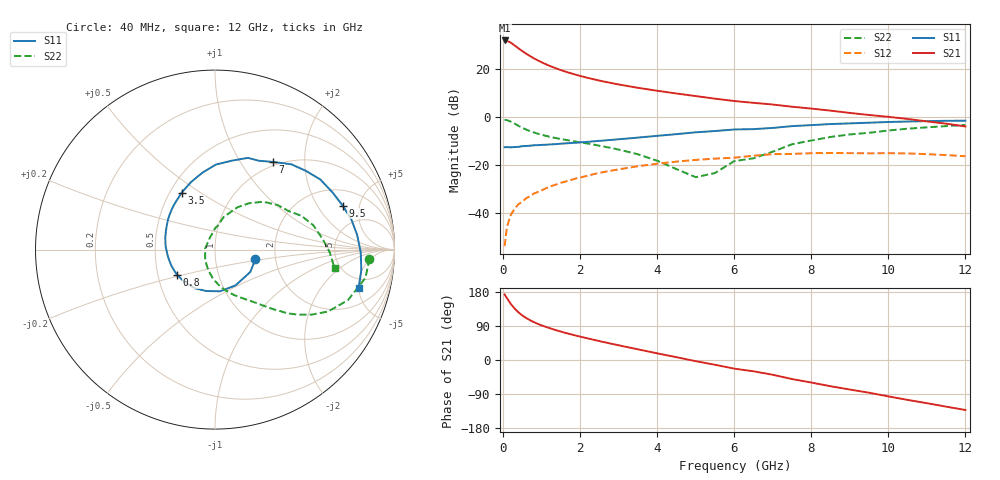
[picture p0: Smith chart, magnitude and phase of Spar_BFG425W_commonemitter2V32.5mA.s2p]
! Filename: 232bfg425.001
! BFG425W Field C1
! V1=8.734E-001V,V2=2.000E+000V, I1=4.905E-004A, I2=3.245E-002A
# GHz  S  MA  R 50
!  S11  S21  S12  S22
!Freq(GHz)  Mag  Ang  Mag  Ang  Mag  Ang  Mag  Ang
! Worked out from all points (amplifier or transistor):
!   44 points, 40 MHz to 12 GHz, reference 50 ohm
!   highest |S21| = 31.8 dB at 40 MHz (marker M1)
!   |S21| within 3 dB of that: start of sweep to 376.2 MHz
!   unconditionally stable (mu >= 1): start of sweep to 68.76 MHz; 867.7 MHz to end of sweep
!   at 700 MHz: K = 0.95, MSG = 29.2 dB, |S12| = -33.2 dB
!   at 2.4 GHz: K = 1.21, MAG = 16.8 dB, |S12| = -23.7 dB
!   at 12 GHz: K = 1.39, MAG = 2.5 dB, |S12| = -16.5 dB
!   S11 on the Smith chart (normalised r, x): 40 MHz: 1.57, -0.17; 800 MHz: 0.63, -0.19; 3.5 GHz: 0.57, +0.42; 7 GHz: 0.94, +1.40; 9.5 GHz: 3.02, +3.41; 12 GHz: 3.72, -5.03
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0.04  0.231 -13.1  39.05 172.9  0.002 76.8  0.862 -3.3
0.1  0.233 -32.3  38.28 163.2  0.005 80.0  0.853 -10.6
0.2  0.23 -60.3  35.17 148.0  0.009 74.2  0.793 -20.7
0.3  0.234 -83.3  30.69 135.7  0.012 70.6  0.719 -28.7
0.4  0.236 -102.2  26.76 125.8  0.015 68.0  0.647 -34.1
0.5  0.243 -117.6  23.43 117.3  0.017 65.8  0.589 -38.0
0.6  0.246 -129.1  20.68 110.7  0.02 64.8  0.541 -41.1
0.7  0.249 -138.4  18.45 105.0  0.022 63.8  0.501 -43.3
0.8  0.254 -146.6  16.58 99.9  0.025 63.3  0.471 -45.2
1  0.259 -159.8  13.69 91.4  0.029 61.9  0.421 -48.5
1.3  0.267 -174.9  10.78 81.0  0.037 59.8  0.37 -52.9
1.7  0.281 169.6  8.344 69.4  0.047 56.3  0.322 -58.8
2.2  0.3 153.6  6.473 56.9  0.059 50.6  0.276 -66.9
2.8  0.329 137.2  5.066 43.2  0.075 42.8  0.224 -78.0
3.5  0.368 120.4  4.019 28.2  0.093 32.8  0.165 -93.4
4.5  0.434 99.3  3.059 7.4  0.116 17.3  0.081 -132.5
6.5  0.552 63.7  1.953 -29.8  0.154 -11.5  0.136 82.8
7  0.585 56.7  1.8 -39.0  0.166 -19.3  0.187 75.3
8.5  0.705 33.6  1.342 -69.3  0.176 -47.9  0.379 44.7
9.5  0.752 19.1  1.09 -86.4  0.173 -64.1  0.463 27.7
10.5  0.796 5.9  0.9 -105.3  0.172 -82.2  0.564 14.0
12  0.829 -14.8  0.628 -131.9  0.15 -111.0  0.674 -8.9
